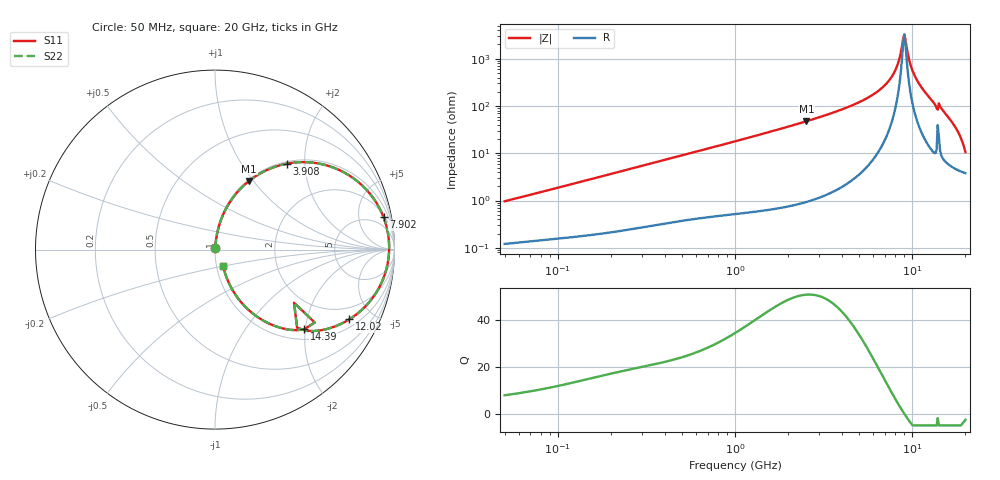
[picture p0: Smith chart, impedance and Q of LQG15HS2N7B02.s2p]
!Murata Part Number: LQG15HS2N7B02
!These Parameters are Measured in Series Mode Connection
!  o--[Z]--o
!Port1  Port2
!  o-------o
!Freq. Start=50[MHz] Stop=20[GHz], 401[Steps]
# Hz S RI R 50
!Freq.(Hz) S11(Real) S11(Imag) S21(Real) S21(Imag) S12(Real) S12(Imag) S22(Real) S22(Imag)
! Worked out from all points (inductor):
!   401 points, 50 MHz to 20 GHz, reference 50 ohm
!   read as one part in series: L = 3.02 nH near 51.52 MHz
!   highest Q = 50.9 at 2.531 GHz (marker M1), where L = 2.99 nH
!   self-resonance near 8.907 GHz
!   S11 on the Smith chart (normalised r, x): 50 MHz: 1.00, +0.02; 3.908 GHz: 1.04, +1.63; 7.902 GHz: 2, +10; 12.02 GHz: 1.35, -3.64; 14.39 GHz: 1.23, -1.97; 20 GHz: 1.08, -0.20
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5e7  0.0013 0.00956  0.9987 -0.00956  0.9987 -0.00956  0.0013 0.00956
1.364002e8  0.0024 0.0251  0.9976 -0.0251  0.9976 -0.0251  0.0024 0.0251
3.721004e8  0.00758 0.0666  0.9924 -0.0666  0.9924 -0.0666  0.00758 0.0666
1e9  0.0357 0.1715  0.9643 -0.1715  0.9643 -0.1715  0.0357 0.1715
2.531158e9  0.1895 0.3822  0.8105 -0.3822  0.8105 -0.3822  0.1895 0.3822
2.728004e9  0.2167 0.4023  0.7833 -0.4023  0.7833 -0.4023  0.2167 0.4023
3.908127e9  0.4016 0.4791  0.5984 -0.4791  0.5984 -0.4791  0.4016 0.4791
5.856089e9  0.72 0.4297  0.28 -0.4297  0.28 -0.4297  0.72 0.4297
7.442007e9  0.9065 0.2487  0.0935 -0.2487  0.0935 -0.2487  0.9065 0.2487
7.901521e9  0.9389 0.1807  0.0611 -0.1807  0.0611 -0.1807  0.9389 0.1807
8.264682e9  0.9567 0.1242  0.0433 -0.1242  0.0433 -0.1242  0.9567 0.1242
8.774992e9  0.9693 0.0424  0.0307 -0.0424  0.0307 -0.0424  0.9693 0.0424
9.041845e9  0.9702 -0.000624  0.0298 0.000624  0.0298 0.000624  0.9702 -0.000624
9.178299e9  0.9692 -0.0225  0.0308 0.0225  0.0308 0.0225  0.9692 -0.0225
9.745021e9  0.9541 -0.1117  0.0459 0.1117  0.0459 0.1117  0.9541 -0.1117
1.019291e10  0.9306 -0.1785  0.0694 0.1785  0.0694 0.1785  0.9306 -0.1785
1.201863e10  0.7493 -0.3881  0.2507 0.3881  0.2507 0.3881  0.7493 -0.3881
1.354865e10  0.5136 -0.4531  0.4864 0.4531  0.4864 0.4531  0.5136 -0.4531
1.438523e10  0.4955 -0.4444  0.5045 0.4444  0.5045 0.4444  0.4955 -0.4444
1.527346e10  0.3558 -0.4332  0.6442 0.4332  0.6442 0.4332  0.3558 -0.4332
1.747767e10  0.1475 -0.2955  0.8525 0.2955  0.8525 0.2955  0.1475 -0.2955
2e10  0.0453 -0.0905  0.9547 0.0905  0.9547 0.0905  0.0453 -0.0905
